(* Logix 5000 AddOnInstructionDefinition export Banner_S15C_MGN_Param_v4; software revision 33.00; part 2 of 2 *)
(* tags used below, declared in another part *)
   S15C : Banner_S15C_MGN_v4;
   Port_Data : Banner_IOL_Port_v4;
   Port : DINT;
   Local_Control : DINT;
   Command_Being_Processed : BOOL;
   Index_Write_Inprocess : INT;
   Update_Archive : BOOL;
   Inprocess_Index : DINT;
   WRS_Index3 : SINT;
   WRS_Index4 : SINT;
(* Banner_S15C_MGN_Param_v4, continued *)

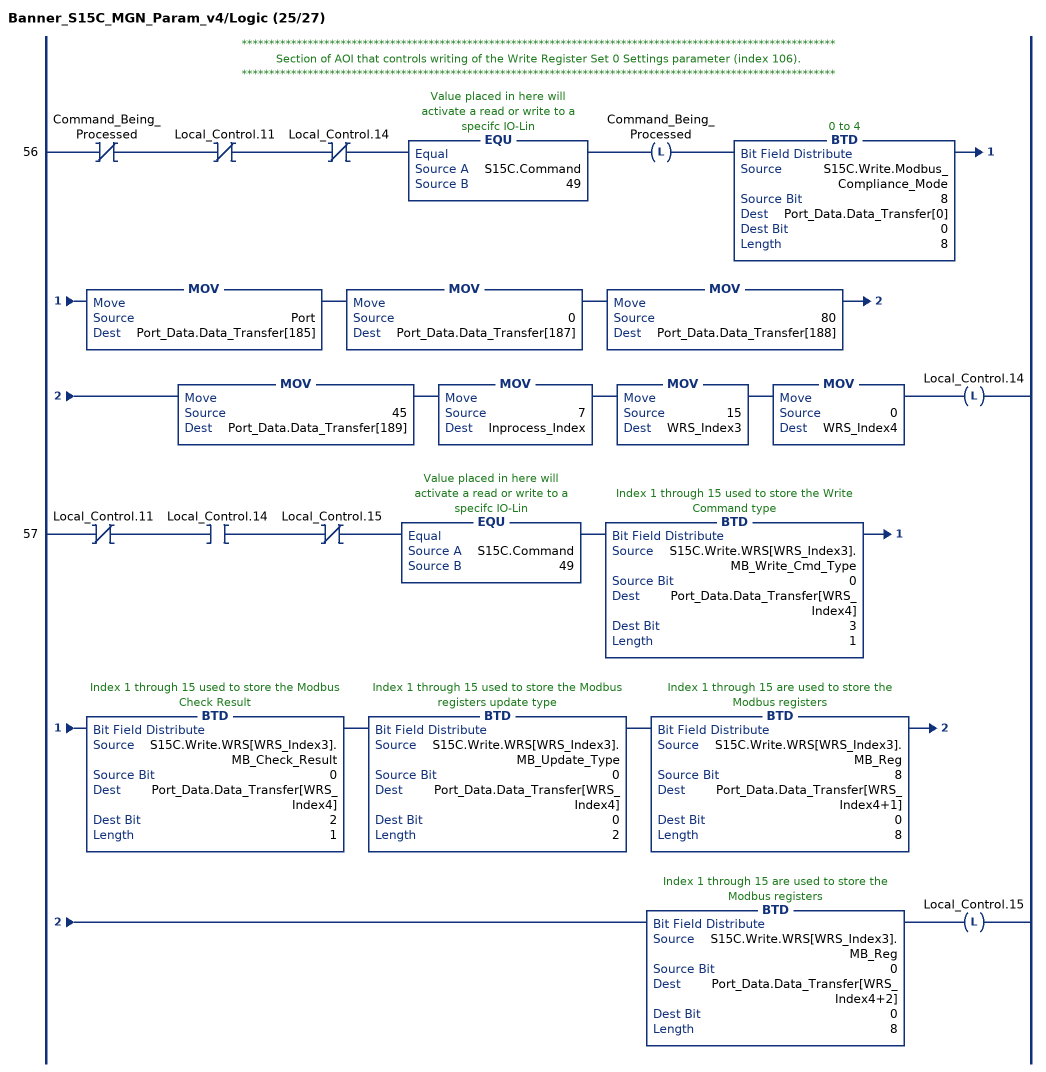
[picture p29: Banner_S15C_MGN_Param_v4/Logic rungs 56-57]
   // ************************************************************************************************************
   // Section of AOI that controls writing of the Write Register Set 0 Settings parameter (index 106).
   // ************************************************************************************************************
   56: XIO(Command_Being_Processed)XIO(Local_Control.11)XIO(Local_Control.14)EQU(S15C.Command,49)OTL(Command_Being_Processed)BTD(S15C.Write.Modbus_Compliance_Mode,8,Port_Data.Data_Transfer[0],0,8)MOV(Port,Port_Data.Data_Transfer[185])MOV(0,Port_Data.Data_Transfer[187])MOV(80,Port_Data.Data_Transfer[188])MOV(45,Port_Data.Data_Transfer[189])MOV(7,Inprocess_Index)MOV(15,WRS_Index3)MOV(0,WRS_Index4)OTL(Local_Control.14);
   57: XIO(Local_Control.11)XIC(Local_Control.14)XIO(Local_Control.15)EQU(S15C.Command,49)BTD(S15C.Write.WRS[WRS_Index3].MB_Write_Cmd_Type,0,Port_Data.Data_Transfer[WRS_Index4],3,1)BTD(S15C.Write.WRS[WRS_Index3].MB_Check_Result,0,Port_Data.Data_Transfer[WRS_Index4],2,1)BTD(S15C.Write.WRS[WRS_Index3].MB_Update_Type,0,Port_Data.Data_Transfer[WRS_Index4],0,2)BTD(S15C.Write.WRS[WRS_Index3].MB_Reg,8,Port_Data.Data_Transfer[WRS_Index4+1],0,8)BTD(S15C.Write.WRS[WRS_Index3].MB_Reg,0,Port_Data.Data_Transfer[WRS_Index4+2],0,8)OTL(Local_Control.15);
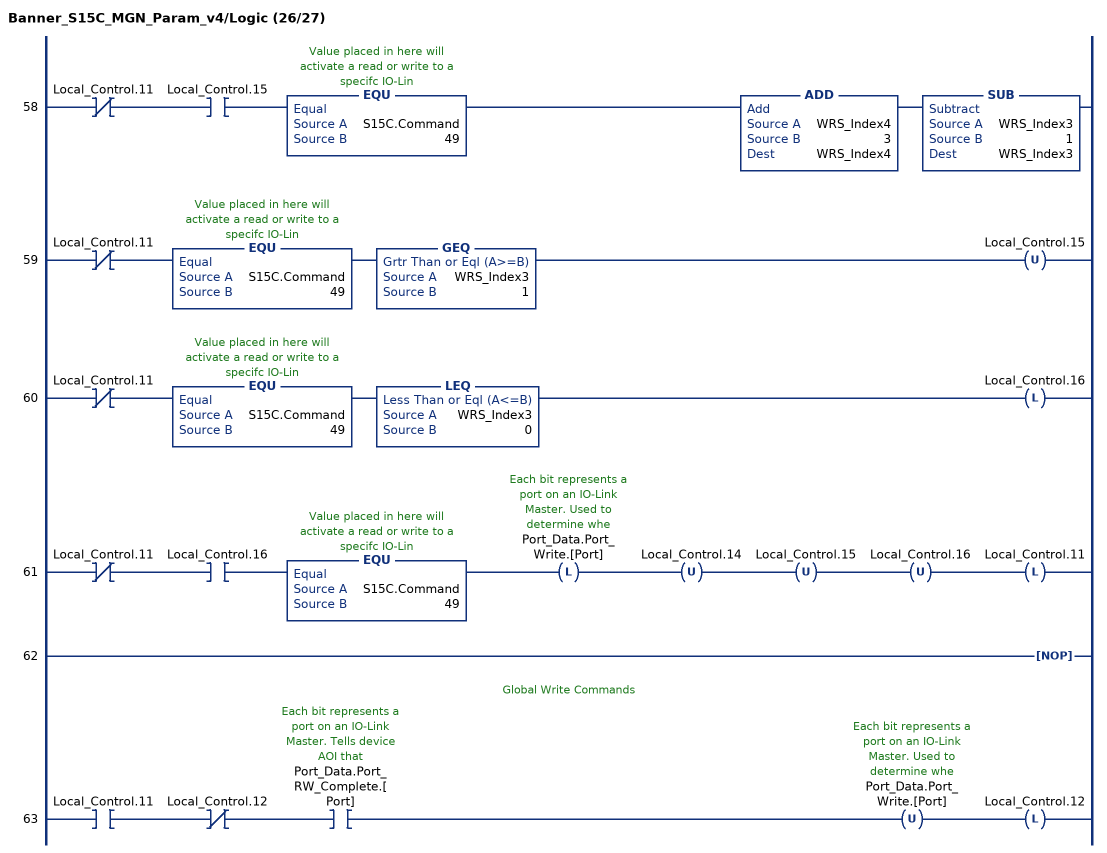
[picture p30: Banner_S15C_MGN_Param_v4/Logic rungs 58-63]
   58: XIO(Local_Control.11)XIC(Local_Control.15)EQU(S15C.Command,49)ADD(WRS_Index4,3,WRS_Index4)SUB(WRS_Index3,1,WRS_Index3);
   59: XIO(Local_Control.11)EQU(S15C.Command,49)GEQ(WRS_Index3,1)OTU(Local_Control.15);
   60: XIO(Local_Control.11)EQU(S15C.Command,49)LEQ(WRS_Index3,0)OTL(Local_Control.16);
   61: XIO(Local_Control.11)XIC(Local_Control.16)EQU(S15C.Command,49)OTL(Port_Data.Port_Write.[Port])OTU(Local_Control.14)OTU(Local_Control.15)OTU(Local_Control.16)OTL(Local_Control.11);
   62: NOP();
   // Global Write Commands
   63: XIC(Local_Control.11)XIO(Local_Control.12)XIC(Port_Data.Port_RW_Complete.[Port])OTU(Port_Data.Port_Write.[Port])OTL(Local_Control.12);
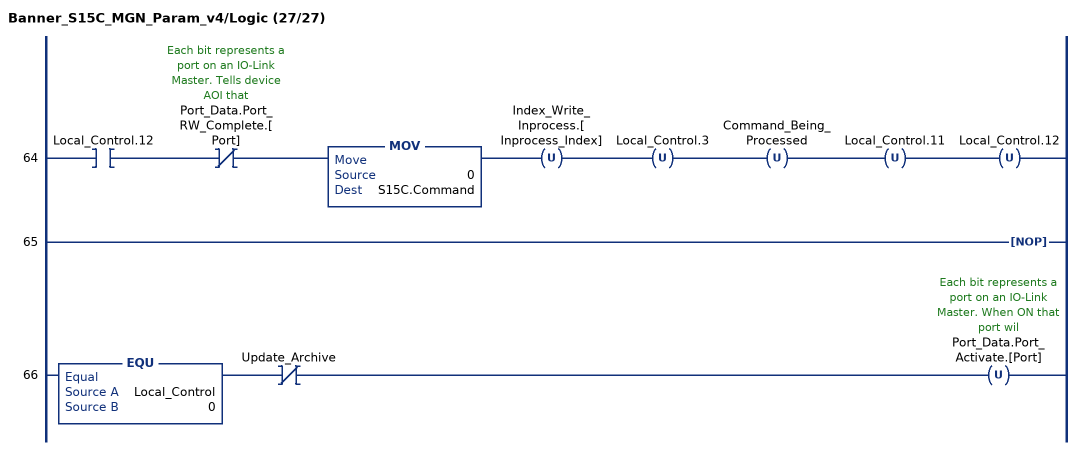
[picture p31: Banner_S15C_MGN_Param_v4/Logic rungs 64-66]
   64: XIC(Local_Control.12)XIO(Port_Data.Port_RW_Complete.[Port])MOV(0,S15C.Command)OTU(Index_Write_Inprocess.[Inprocess_Index])OTU(Local_Control.3)OTU(Command_Being_Processed)OTU(Local_Control.11)OTU(Local_Control.12);
   65: NOP();
   66: EQU(Local_Control,0)XIO(Update_Archive)OTU(Port_Data.Port_Activate.[Port]);
END_ROUTINE
END_ADD_ON_INSTRUCTION
